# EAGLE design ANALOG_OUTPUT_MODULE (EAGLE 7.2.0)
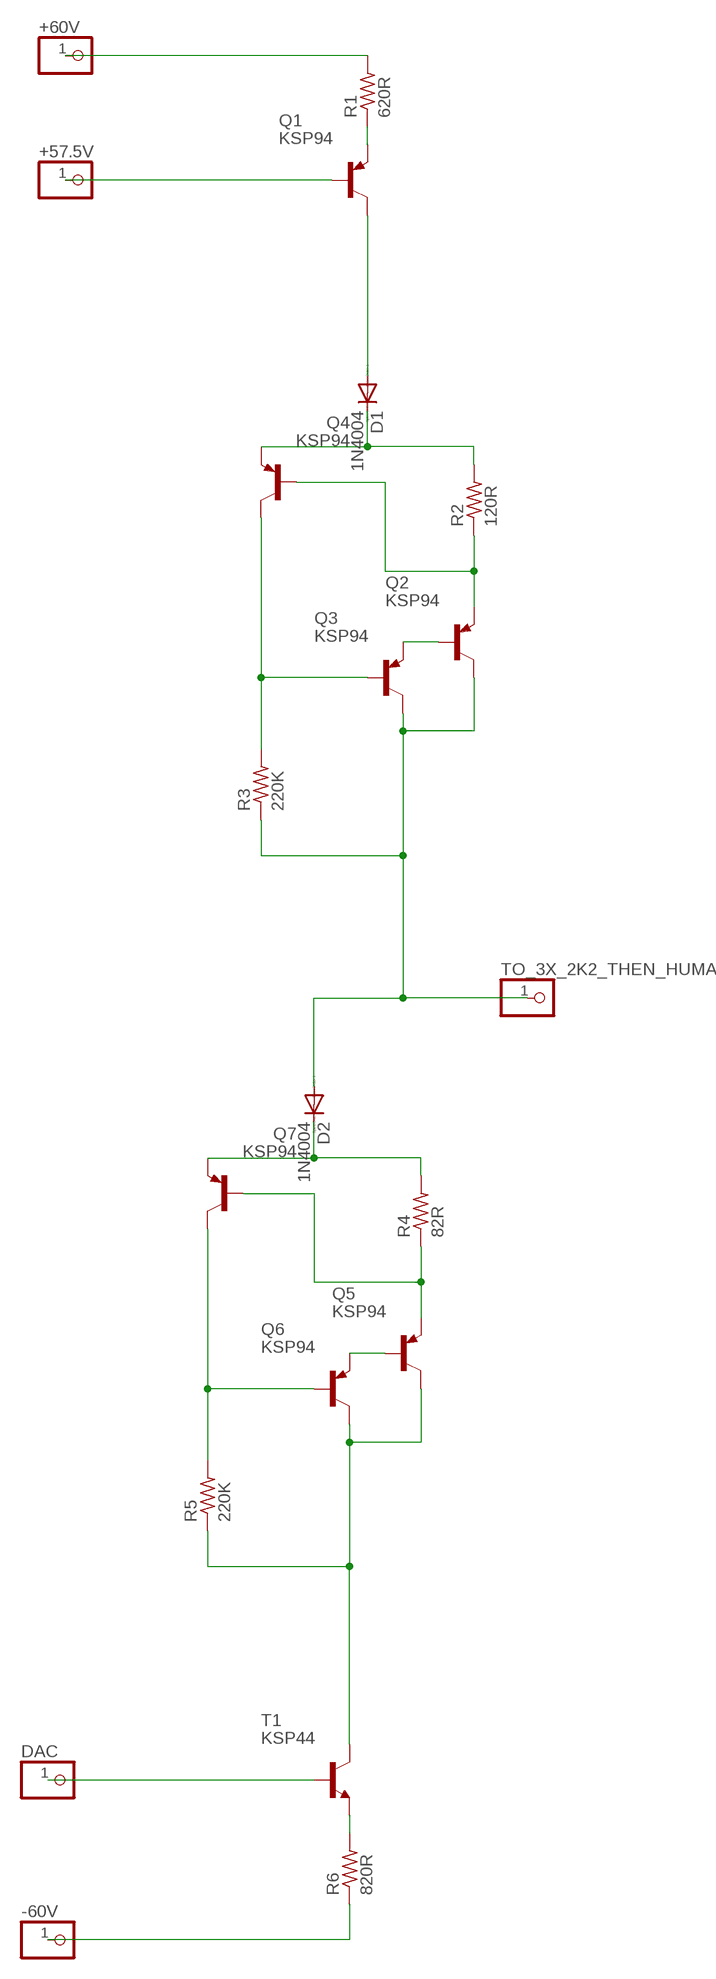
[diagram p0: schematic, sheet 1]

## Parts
+57.5V  PINHD-1X1  [1X01]
+60V  PINHD-1X1  [1X01]
-60V  PINHD-1X1  [1X01]
D1  1N4004  [DO41-10]
D2  1N4004  [DO41-10]
DAC  PINHD-1X1  [1X01]
Q1  KSP94  MPSA56  [TO92-CBE]
Q2  KSP94  MPSA56  [TO92-CBE]
Q3  KSP94  MPSA56  [TO92-CBE]
Q4  KSP94  MPSA56  [TO92-CBE]
Q5  KSP94  MPSA56  [TO92-CBE]
Q6  KSP94  MPSA56  [TO92-CBE]
Q7  KSP94  MPSA56  [TO92-CBE]
R1  620R  R-US_0207/10  [0207/10]
R2  120R  R-US_0207/10  [0207/10]
R3  220K  R-US_0207/10  [0207/10]
R4  82R  R-US_0207/10  [0207/10]
R5  220K  R-US_0207/10  [0207/10]
R6  820R  R-US_0207/10  [0207/10]
T1  KSP44  MPSA06-NPN-TO92-EBC  [TO92-EBC]
TO_3X_2K2_THEN_HUMAN  PINHD-1X1  [1X01]

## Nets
N$1: +60V.1 R1.2
N$2: Q1.E R1.1
N$3: +57.5V.1 Q1.B
N$4: DAC.1 T1.B
N$5: -60V.1 R6.1
N$6: D1.C Q4.E R2.2
N$7: D1.A Q1.C
N$8: Q2.E Q4.B R2.1
N$9: Q2.B Q3.E
N$10: Q3.B Q4.C R3.2
N$11: D2.A Q2.C Q3.C R3.1 TO_3X_2K2_THEN_HUMAN.1
N$12: D2.C Q7.E R4.2
N$13: R6.2 T1.E
N$14: Q5.E Q7.B R4.1
N$15: Q5.B Q6.E
N$16: Q6.B Q7.C R5.2
N$17: Q5.C Q6.C R5.1 T1.C

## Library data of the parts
+57.5V +60V -60V DAC TO_3X_2K2_THEN_HUMAN = pinhead:PINHD-1X1: PIN HEADER
D1 D2 = diode:1N4004: DIODE
Q1-Q7 = transistor-pnp:MPSA56*: PNP Transistror Source: http://www.fairchildsemi.com/ds/MM/MMBTA56.pdf
R1-R6 = rcl:R-US_: RESISTOR, American symbol
T1 = transistor:*-NPN-: NPN Transistror BF959 corrected 2008.03.06

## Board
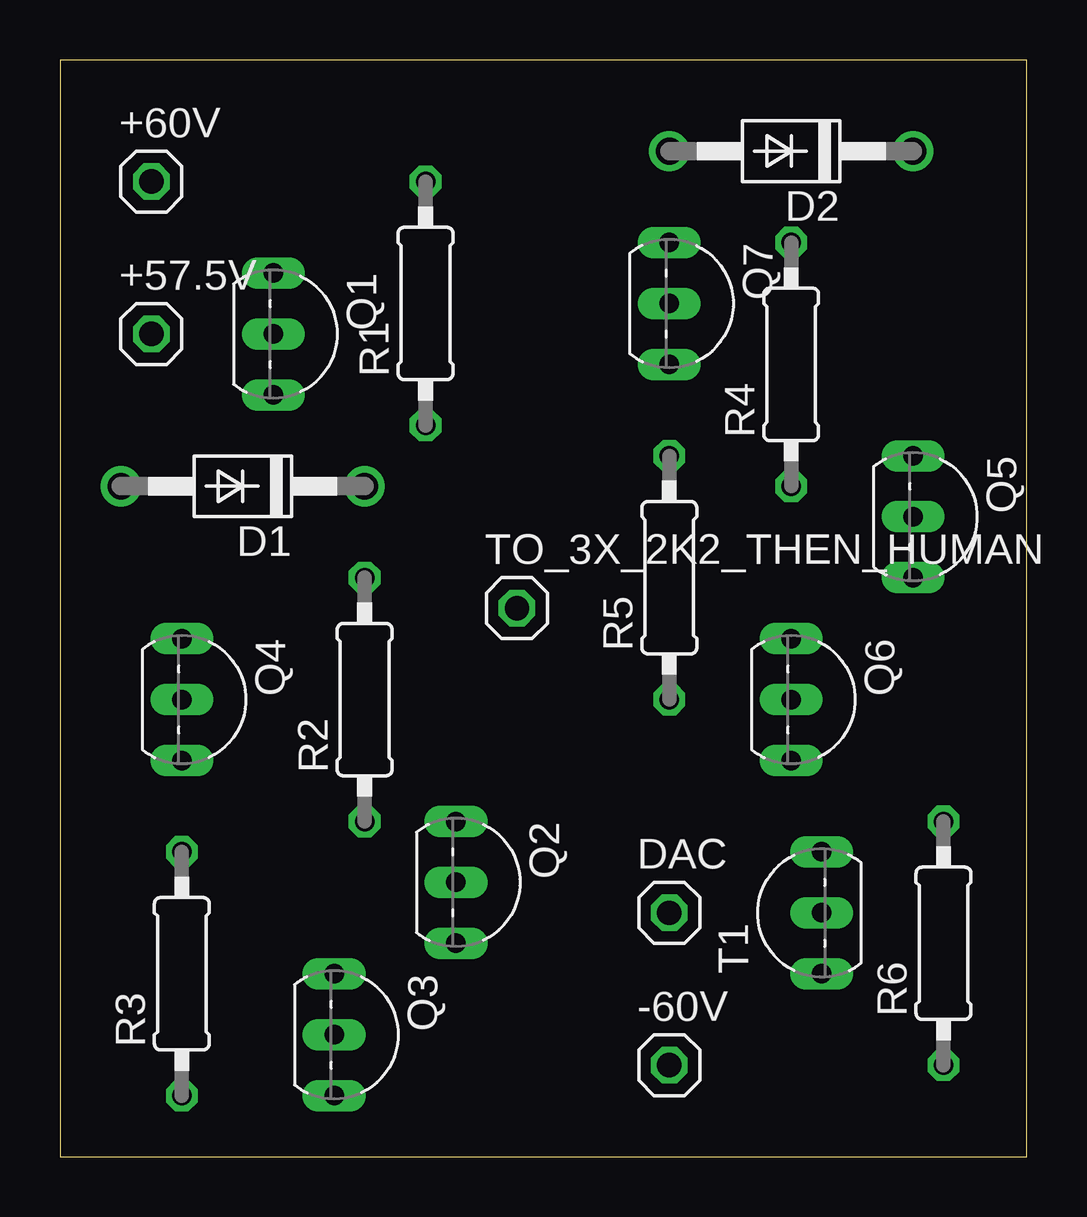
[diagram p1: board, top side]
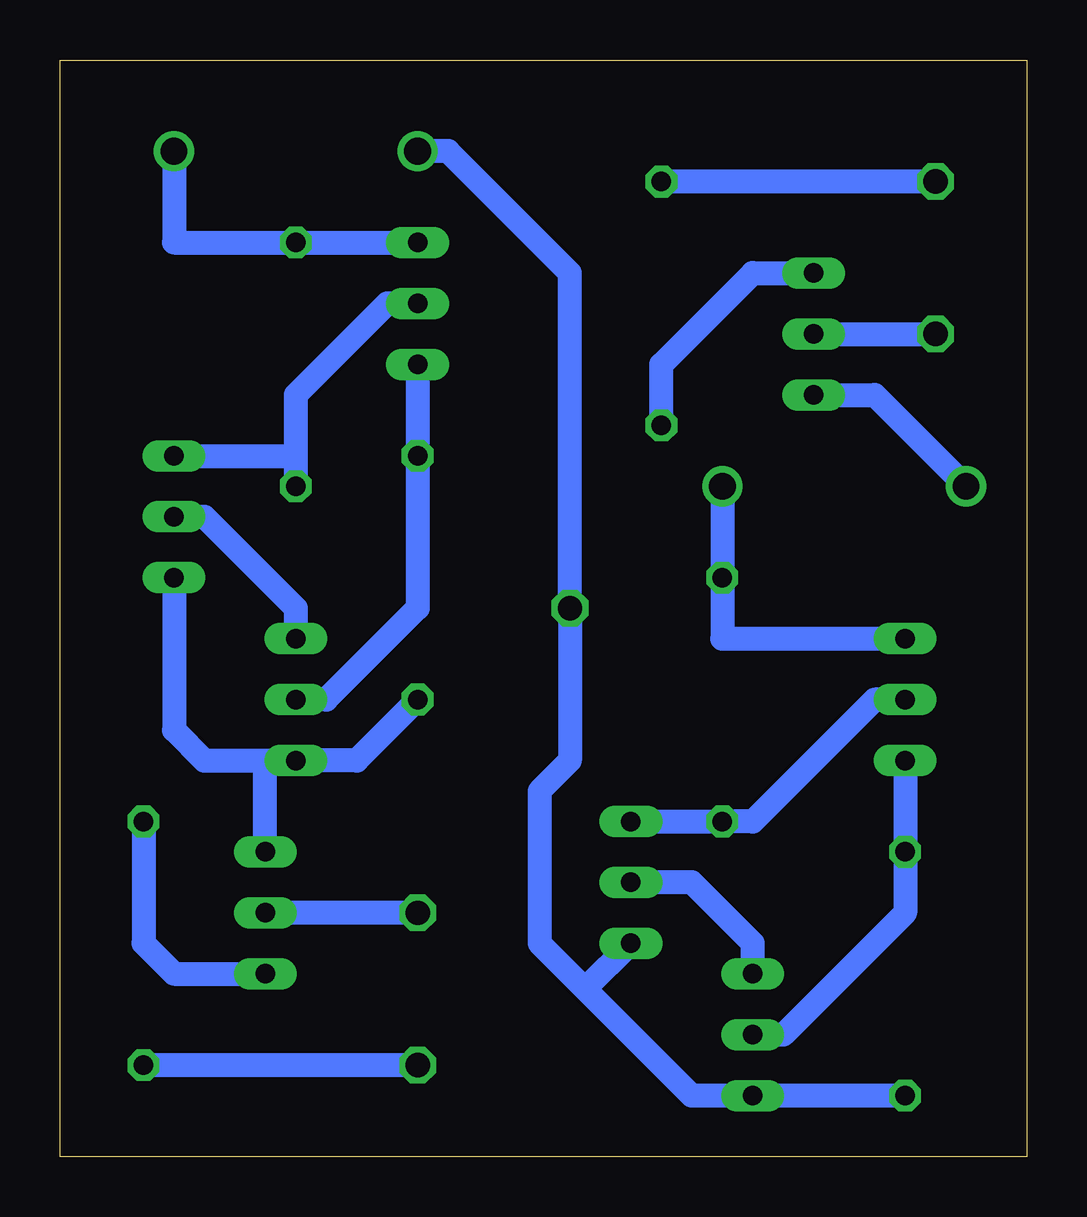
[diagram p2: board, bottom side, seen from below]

Size 40.31 x 45.71 mm. Coordinates in mm from the lower left corner, seen from the top.
Outline: 0,0 40.31,0 40.31,45.71 0,45.71 0,0
Copper layers (1*16): Top 0.035mm / dielectric 1.5mm / Bottom 0.035mm
Design rules "default": minimum track width 10mil, minimum drill 24mil, track to track 8mil, track to pad 8mil, pad to pad 8mil, via to via 8mil, smd to smd 8mil, copper to edge 40mil, drill to drill 8mil, minimum pad ring 10mil, minimum via ring 8mil, stop-mask expansion 4mil, vias tented up to drill 0mil, thermal gap 10mil

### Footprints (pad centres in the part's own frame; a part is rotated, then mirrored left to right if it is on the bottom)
1X01 = drill 1.016 octagon: 1 0,0
DO41-10 = drill 1.118: A 5.08,0; C -5.08,0
TO92-CBE = drill 0.813 long: B 0,0; C 2.54,0; E -2.54,0
0207/10 = drill 0.813 octagon: 1 -5.08,0; 2 5.08,0
TO92-EBC = drill 0.813 long: B 0,-1.27; C 2.54,-1.27; E -2.54,-1.27

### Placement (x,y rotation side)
+57.5V  3.81,34.29 0 top
+60V  3.81,40.64 0 top
-60V  25.4,3.81 0 top
D1  7.62,27.94 180 top
D2  30.48,41.91 180 top
DAC  25.4,10.16 0 top
Q1  8.89,34.29 270 top
Q2  16.51,11.43 270 top
Q3  11.43,5.08 270 top
Q4  5.08,19.05 270 top
Q5  35.56,26.67 270 top
Q6  30.48,19.05 270 top
Q7  25.4,35.56 270 top
R1  15.24,35.56 90 top
R2  12.7,19.05 90 top
R3  5.08,7.62 90 top
R4  30.48,33.02 90 top
R5  25.4,24.13 90 top
R6  36.83,8.89 90 top
T1  30.48,10.16 90 top
TO_3X_2K2_THEN_HUMAN  19.05,22.86 0 top

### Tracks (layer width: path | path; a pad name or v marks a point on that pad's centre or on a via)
N$1
  Bottom 1: +60V.1 R1.2
N$2
  Bottom 1: R1.1 15.24,33.02 11.43,36.83 Q1.E
N$3
  Bottom 1: Q1.B +57.5V.1
N$4
  Bottom 1: DAC.1 T1.B
N$5
  Bottom 1: -60V.1 R6.1
N$6
  Bottom 1: D1.C R2.2 12.7,21.59 Q4.E
N$7
  Bottom 1: Q1.C 6.35,31.75 D1.A
N$8
  Bottom 1: Q4.B 6.35,19.05 11.43,13.97 R2.1 Q2.E
N$9
  Bottom 1: Q3.E 11.43,8.89 13.97,11.43 Q2.B
N$10
  Bottom 1: Q4.C R3.2 5.08,10.16 10.16,5.08 Q3.B
N$11
  Bottom 1: R3.1 Q3.C 13.97,2.54 18.41,6.99 | 18.41,6.99 20.32,8.89 20.32,15.24 19.05,16.51 TO_3X_2K2_THEN_HUMAN.1 19.05,36.83 24.13,41.91 D2.A | Q2.C 18.41,6.99
N$12
  Bottom 1: D2.C 35.56,38.1 R4.2 Q7.E
N$13
  Bottom 1: T1.E 35.56,7.62 36.83,8.89 R6.2
N$14
  Bottom 1: Q7.B 26.67,35.56 30.48,31.75 30.48,29.21 | 30.48,29.21 R4.1 | Q5.E 30.48,29.21
N$15
  Bottom 1: Q5.B 34.29,26.67 30.48,22.86 Q6.E
N$16
  Bottom 1: Q7.C R5.2 25.4,22.86 29.21,19.05 Q6.B
N$17
  Bottom 1: Q5.C 35.56,17.78 34.29,16.51 31.75,16.51 | 31.75,16.51 Q6.C 27.94,16.51 R5.1 | T1.C 31.75,16.51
